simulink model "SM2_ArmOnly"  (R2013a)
settings: Solver=ode45  StartTime=0  StopTime=2  FixedStep=1e-4  RelTol=1e-3  AbsTol=1e-4
PreLoadFcn:
  | warning('off','sm:sli:setup:compile:LocalSolverNotSupported')
InitFcn:
  | if(~Model.ModelUpdate)
  |  [~]=SM2_ArmOnly_ConstrFnc(0,Model);
  |  SimParam.IC = SM2_InitCondConstrFnc(RawParam,IC);
  |  Model.ModelUpdate=1;
  | end
model workspace (MAT data in the model file):
  handle : class17 (value not decoded)
  handle : class17 (value not decoded)
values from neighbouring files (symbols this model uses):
  m = v*BEAM.rho    [FlexBeamModelConstruct2.m]    (also in FlexBeamModelConstruct3.m = BEAM.rho*v; FlexBeam_1D_Construct.m = REF.m/REF.l*a.*(linspace(1-OPT.MassBiais+1e-6,1+OPT.MassBiai; FlexBeam_3D_Construct.m = REF.m/REF.l*a.*(linspace(1-OPT.MassBiais+1e-6,1+OPT.MassBiai; FreeFlexBeam_3D_Construct.m = REF.m/REF.l*a.*tmp2)
  RawParam = RobotParamGather(ParamLib)    [DeltaModelMain_v2.m]    (also in main_TimeSimulation.m; MGI.m = y)
undefined symbols (not defined in the file or in its folder): kg
libraries: sm_lib x3, SM2_ArmPartsLib x1, SM2_MotorPartsLib x1, SM2_FramePartsLib x1

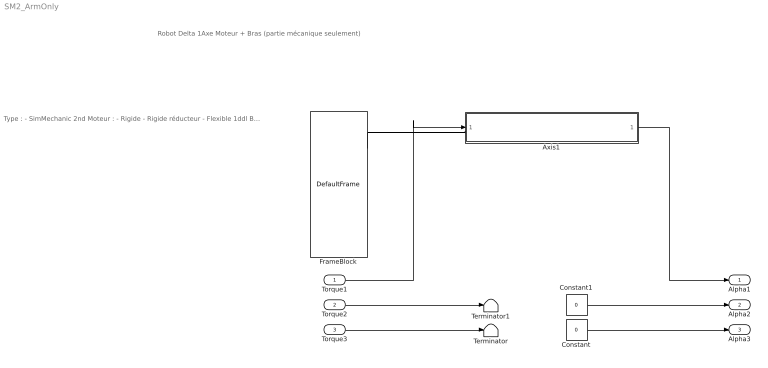
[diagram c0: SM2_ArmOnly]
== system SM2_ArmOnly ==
  note: Robot Delta 1Axe Moteur + Bras (partie mécanique seulement)
  note: Type : - SimMechanic 2nd Moteur : - Rigide - Rigide réducteur - Flexible 1ddl Bras : - Rigide - Flexible 3ddl (2,3,4 seg.)
  Torque1 : Inport
  Torque2 : Inport  Port=2
  Torque3 : Inport  Port=3
  Axis1 : Subsystem
  Constant : Constant  Value=0
  Constant1 : Constant  Value=0
  FrameBlock : SM2_FramePartsLib/DefaultFrame
  Terminator : Terminator
  Terminator1 : Terminator
  Alpha1 : Outport
  Alpha2 : Outport  Port=2
  Alpha3 : Outport  Port=3
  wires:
  Axis1/1(Alpha) -> Alpha1/1
  Constant/1 -> Alpha3/1
  Torque3/1 -> Terminator/1
  Torque2/1 -> Terminator1/1
  Constant1/1 -> Alpha2/1
  Torque1/1 -> Axis1/1(Torque)
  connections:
  FrameBlock/RConn1 -- Axis1/LConn1

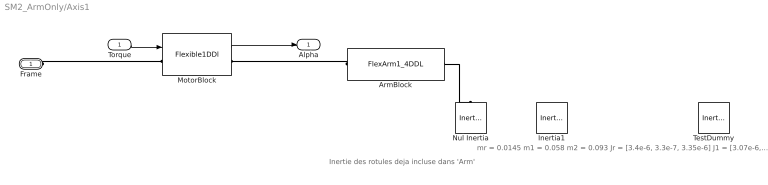
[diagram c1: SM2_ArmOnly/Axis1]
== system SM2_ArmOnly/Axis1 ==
  note: Inertie des rotules deja incluse dans 'Arm'
  note: mr = 0.0145 m1 = 0.058 m2 = 0.093 Jr = [3.4e-6, 3.3e-7, 3.35e-6] J1 = [3.07e-6, 4.18e-6, 5.04e-6] J2 = [6.29e-6, 10.2e-6, 10.2e-6]
  Torque : Inport
  ArmBlock : SM2_ArmPartsLib/FlexArm1_4DDL  VariantControl=armVarFlex1_4ddl
  Inertia1 : sm_lib/Body Elements/Inertia  Commented=on  InertiaType=Custom  Mass=0.083  MassUnits=kg  CenterOfMass=[0 0 0]  CenterOfMassUnits=m  MomentsOfInertia=[6.29e-6, 10.2e-6, 10.2e-6]  MomentsOfInertiaUnits=kg*m^2  ProductsOfInertia=[0 0 0]  ProductsOfInertiaUnits=kg*m^2  BlockFunction=simmechanics.library.body_elements.inertia
  MotorBlock : SM2_MotorPartsLib/Flexible1DDl  VariantControl=motorVarFlex1
  Nul Inertia : sm_lib/Body Elements/Inertia  InertiaType=Custom  Mass=1e-5  MassUnits=kg  CenterOfMass=[0 0 0]  CenterOfMassUnits=m  MomentsOfInertia=[1e-8 1e-8 1e-8]  MomentsOfInertiaUnits=kg*m^2  ProductsOfInertia=[0 0 0]  ProductsOfInertiaUnits=kg*m^2  BlockFunction=simmechanics.library.body_elements.inertia
  TestDummy : sm_lib/Body Elements/Inertia  Commented=on  InertiaType=Custom  Mass=0.0145  MassUnits=kg  CenterOfMass=[0 0 0]  CenterOfMassUnits=m  MomentsOfInertia=[3.4e-6, 3.3e-7, 3.35e-6]  MomentsOfInertiaUnits=kg*m^2  ProductsOfInertia=[0 0 0]  ProductsOfInertiaUnits=kg*m^2  BlockFunction=simmechanics.library.body_elements.inertia
  Frame : PMIOPort  Port=1  Side=Left
  Alpha : Outport
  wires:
  Torque/1 -> MotorBlock/1
  MotorBlock/1 -> Alpha/1
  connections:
  Frame/RConn1 -- MotorBlock/LConn1
  ArmBlock/LConn1 -- MotorBlock/RConn1
  ArmBlock/RConn1 -- Nul Inertia/RConn1
